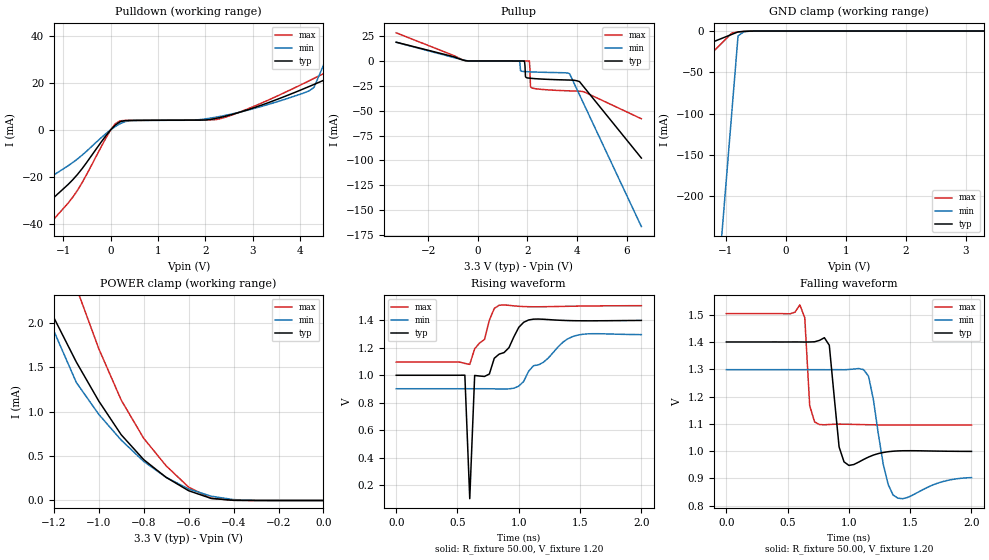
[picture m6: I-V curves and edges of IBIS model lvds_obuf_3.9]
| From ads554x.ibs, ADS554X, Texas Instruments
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|   Model lvds_obuf_3.9
[Model]   lvds_obuf_3.9
Model_type   3-state
Polarity   Non-Inverting
Enable   Active-High
Vmeas =   1.2000V
Cref =   5.0000pF
Rref = 50.0000
Vref =   1.2000V
C_comp   2.13pF   1.93pF   2.33pF
[Temperature Range]   27.00   125   -40.00
[Voltage Range]   3.30V   3.00V   3.60V
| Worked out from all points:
|   slope of the pulldown table from 0 to 0.495 V, typ, clamps not added: 123 ohm
|   GND clamp passes 1 mA (typ) near -0.79 V on its own axis
|   POWER clamp passes 1 mA (typ) near -0.97 V on its own axis
|   rising waveform, R_fixture 50.00, V_fixture 1.20: 20-80 % time 198ps typ, 279ps min, 136ps max; typ from 0.999 V to 1.4 V
|   falling waveform, R_fixture 50.00, V_fixture 1.20: 20-80 % time 51.6ps typ, 83.6ps min, 30.5ps max; typ from 1.4 V to 0.999 V
[Pulldown]
| voltage   I(typ)   I(min)   I(max)
-3.3V     -67.49mA   -46.56mA   -85.28mA
-2.1V     -45.41mA   -30.96mA   -58.28mA
-1.5V     -34.37mA   -23.16mA   -44.78mA
-800mV    -21.3mA    -13.97mA   -28.72mA
200mV     3.38mA     2.54mA     3.77mA
2.4V      5.6mA      5.99mA     5.16mA
4.3V      19.26mA    18.03mA    21.84mA
4.7V      22.91mA    36.93mA    25.86mA
4.9V      29.14mA    46.38mA    27.9mA
5.1V      48.06mA    55.83mA    30.14mA
5.5V      85.9mA     74.73mA    60.76mA
6.6V      190mA      126.7mA    179.3mA
[Pullup]
| voltage   I(typ)   I(min)   I(max)
-3.3V     18.97mA    18.87mA    28.41mA
-500mV    360uA      560uA      330uA
1.68V     28.88uA    11.39uA    48.96uA
1.72V     27.06uA    -9.697mA   46.62uA
1.88V     13.55uA    -10.57mA   37.22uA
1.92V     -15.65mA   -10.64mA   34.86uA
2.08V     -17.25mA   -10.84mA   -27.96uA
2.12V     -17.34mA   -10.89mA   -25mA
2.16V     -17.43mA   -10.93mA   -26.76mA
3.7V      -19.14mA   -12.67mA   -30.03mA
4.1V      -20.67mA   -33.91mA   -30.35mA
6.6V      -97.67mA   -166.7mA   -58.11mA
[GND_clamp]
| voltage   I(typ)   I(min)   I(max)
-3.3V     -73.53mA   -2.228A    -176.7mA
-1.1V     -9.73mA    -272.6mA   -16.77mA
-1V       -6.83mA    -183.7mA   -9.5mA
-900mV    -3.93mA    -94.8mA    -2.23mA
-800mV    -1.03mA    -5.92mA    -1.19mA
-700mV    -450uA     -730uA     -490uA
3.3V      44.64pA    1.08uA     37.43pA
[POWER_clamp]
| voltage   I(typ)   I(min)   I(max)
-3.3V     247.8mA    491.9mA    558.7mA
-1.3V     2.62mA     3.21mA     3.99mA
-1.2V     2.06mA     1.91mA     3.16mA
-1.1V     1.56mA     1.33mA     2.4mA
-1V       1.12mA     970uA      1.71mA
-900mV    740uA      680uA      1.13mA
-800mV    460uA      440uA      700uA
-700mV    260uA      260uA      390uA
-600mV    110uA      130uA      150uA
-500mV    23.34uA    48.47uA    24.97uA
-400mV    2uA        9.55uA     1.31uA
0V        44.64pA    500pA      43.31pA
[Ramp]
| variable   typ   min   max
dV/dt_r   1.84/71.07p   1.61/0.12n   2.05/47.67p
dV/dt_f   1.67/0.18n   1.55/0.16n   1.71/0.27n
R_load = 1.00k
[Rising Waveform]
R_fixture = 50.00
V_fixture = 1.20
V_fixture_min = 1.10
V_fixture_max = 1.30
| time   V(typ)   V(min)   V(max)
0s        999.4mV    901.2mV    1.096V
560ps     999.9mV    901.2mV    1.086V
600ps     100mV      901.3mV    1.079V
640ps     998mV      901.3mV    1.192V
720ps     990.7mV    901.3mV    1.26V
760ps     1.009V     901.1mV    1.401V
800ps     1.123V     900.4mV    1.486V
1ns       1.349V     920.1mV    1.502V
1.44ns    1.397V     1.282V     1.503V
2ns       1.399V     1.296V     1.506V
[Falling Waveform]
R_fixture = 50.00
V_fixture = 1.20
V_fixture_min = 1.10
V_fixture_max = 1.30
| time   V(typ)   V(min)   V(max)
0s        1.401V     1.299V     1.505V
600ps     1.401V     1.299V     1.537V
640ps     1.401V     1.299V     1.489V
680ps     1.401V     1.299V     1.167V
800ps     1.417V     1.299V     1.097V
920ps     1.016V     1.299V     1.099V
1ns       948mV      1.3V       1.099V
1.16ns    978.7mV    1.275V     1.097V
1.36ns    1V         839.6mV    1.096V
2ns       999.4mV    903.4mV    1.096V
